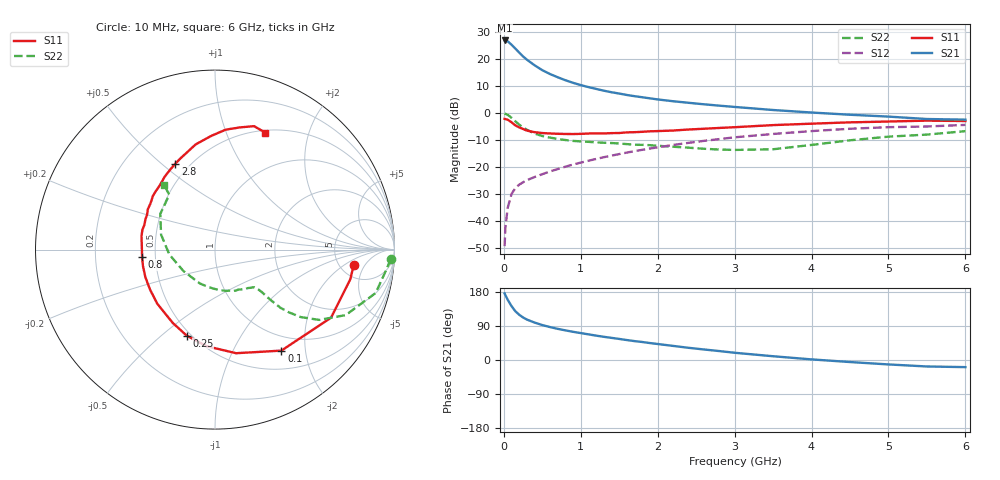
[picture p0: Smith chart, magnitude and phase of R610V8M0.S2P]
! SIEMENS Small Signal Semiconductors
! BFR193
! Si NPN RF Bipolar Junction Transistor in SOT23
! VCE = 10 V  IC = 8 mA
! Common Emitter S-Parameters:  May  1996
# GHz  S  MA  R  50
!  f  S11  S21  S12  S22
! GHz  MAG  ANG  MAG  ANG  MAG  ANG  MAG  ANG
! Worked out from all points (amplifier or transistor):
!   36 points, 10 MHz to 6 GHz, reference 50 ohm
!   highest |S21| = 26.9 dB at 10 MHz (marker M1)
!   |S21| within 3 dB of that: start of sweep to 149.2 MHz
!   unconditionally stable (mu >= 1): 822.4 MHz to 2.081 GHz
!   at 250 MHz: K = 0.56, MSG = 23.3 dB, |S12| = -25.7 dB
!   at 1.4 GHz: K = 1.05, MAG = 10.4 dB, |S12| = -15.8 dB
!   at 6 GHz: K = 0.94, MSG = 1.0 dB, |S12| = -4.4 dB
!   S11 on the Smith chart (normalised r, x): 10 MHz: 6.75, -2.87; 100 MHz: 0.77, -1.58; 250 MHz: 0.47, -0.61; 800 MHz: 0.42, -0.04; 2.8 GHz: 0.42, +0.56; 6 GHz: 0.53, +1.38
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0.01  0.7775 -6.2  22.08 175.7  0.0034 82.2  0.9798 -3.1
0.02  0.772 -12.3  22.08 171.1  0.0075 83.3  0.9638 -6.2
0.05  0.7497 -30.4  21.32 159.1  0.0174 73.5  0.9275 -15.1
0.1  0.6734 -56.7  18.41 142.2  0.0315 64.8  0.8147 -26.6
0.15  0.5891 -78.5  15.6 128.6  0.0406 58.1  0.7005 -34.0
0.2  0.5401 -95.0  13.17 119.4  0.047 55.0  0.6079 -38.2
0.25  0.5046 -108.2  11.16 112.2  0.052 53.2  0.5407 -40.3
0.3  0.4716 -119.9  9.715 106.7  0.0569 53.4  0.489 -41.6
0.4  0.4409 -136.8  7.646 98.7  0.065 53.9  0.4161 -42.2
0.5  0.4249 -148.5  6.211 92.2  0.0734 55.5  0.3736 -42.2
0.6  0.4172 -158.5  5.274 86.9  0.0825 56.9  0.3493 -42.2
0.8  0.4082 -174.4  4.048 78.2  0.101 59.1  0.3154 -43.2
0.9  0.4072 180.0  3.622 74.4  0.1108 60.0  0.3036 -43.8
1.1  0.4164 169.6  3.018 67.7  0.1303 60.8  0.2918 -46.8
1.3  0.4168 160.6  2.59 61.2  0.1516 60.7  0.2806 -50.0
1.6  0.4368 148.9  2.154 52.6  0.1846 59.7  0.2648 -57.0
2.2  0.4727 130.4  1.65 37.2  0.2554 55.2  0.237 -75.4
2.8  0.5278 114.7  1.367 23.6  0.328 48.4  0.2101 -102.7
3.5  0.596 100.4  1.135 9.9  0.4086 38.4  0.2126 -145.9
4.5  0.6704 85.0  0.927 -5.4  0.5099 23.5  0.3117 164.5
5.5  0.7215 72.4  0.773 -17.1  0.5619 7.5  0.3976 129.8
6  0.7093 66.8  0.752 -18.8  0.6012 3.0  0.4604 128.2
